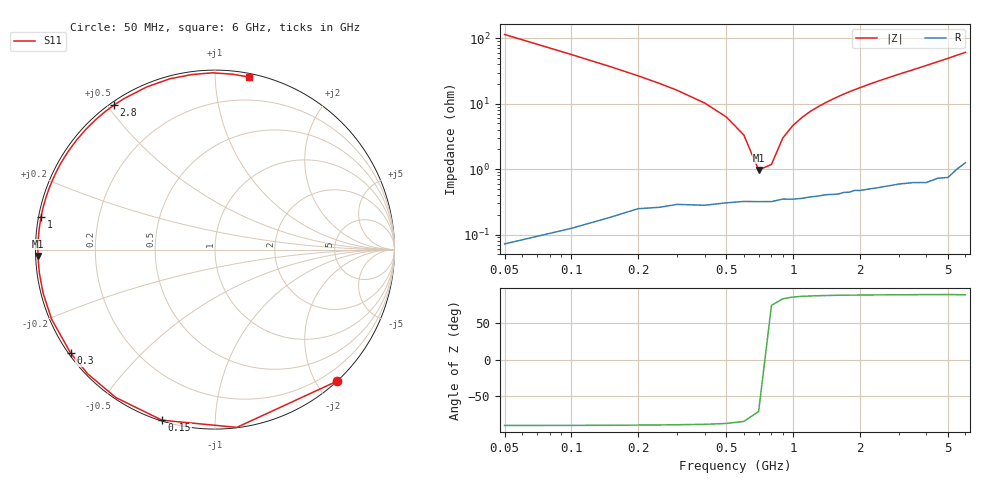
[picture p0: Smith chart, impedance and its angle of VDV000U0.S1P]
! Infineon Technologies  Discrete & RF Semiconductors
! BBY 55-03
! Si Tuning Diode in SOD323
! VR = 0 V
! S-Parameters:  June  1999
# GHz  S  MA  R  50
!  f  S11
! GHz  MAG  ANG
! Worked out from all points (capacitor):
!   34 points, 50 MHz to 6 GHz, reference 50 ohm
!   read as one part to ground: C = 27.7 pF near 50 MHz
!   lowest |Z| = 970 mohm at 700 MHz (marker M1)
!   series resonance near 744.7 MHz, so ESL is about 1.7 nH
!   S11 on the Smith chart (normalised r, x): 50 MHz: 0.00, -2.29; 150 MHz: 0.00, -0.74; 300 MHz: 0.01, -0.32; 1 GHz: 0.01, +0.09; 2.8 GHz: 0.01, +0.52; 6 GHz: 0.03, +1.22
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0.05  0.9995 -47.2
0.1  0.9978 -83.0
0.15  0.9953 -107.2
0.2  0.9923 -123.8
0.25  0.9911 -135.6
0.3  0.9896 -144.4
0.4  0.9893 -156.9
0.5  0.9881 -165.7
0.6  0.9873 -172.4
0.7  0.9874 -177.9
0.8  0.9873 177.4
0.9  0.9862 173.2
1  0.9863 169.4
1.2  0.9854 162.6
1.4  0.9846 156.7
1.6  0.9845 151.2
1.7  0.9838 148.5
2  0.9834 141.4
2.2  0.983 136.9
2.4  0.9828 132.7
2.8  0.9824 124.9
3  0.9822 121.2
3.5  0.9829 112.8
4  0.9845 104.8
4.5  0.9837 97.5
5  0.985 90.8
5.5  0.9821 84.4
6  0.9801 78.7
